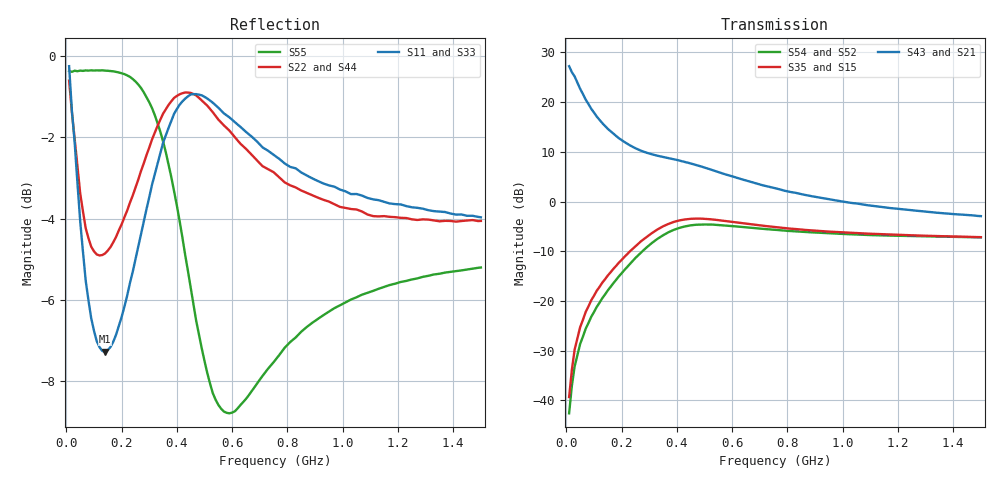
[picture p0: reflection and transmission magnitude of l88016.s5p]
!  1/8/97
!  POLYFET RF DEVICES
!  L88016
!  S PARAMETERS
!  VDS=28V, IDQ=200mA
!AWR Design Environment (2053) Wed Feb 04 14:48:35 2004
!freq-unit  param-type  data-format  keyword  impedance-ohms
# MHz  S  MA  R  50
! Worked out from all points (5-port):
!   150 points, 10 MHz to 1.5 GHz, reference 50 ohm
!   strongest paths, dB at 10 MHz, 380 MHz, 760 MHz, 1.13 GHz, 1.5 GHz:
!     S43: 27.2, 8.6, 2.6, -1.0, -2.9
!     S21: 27.2, 8.6, 2.6, -1.0, -2.9
!     S35: -39.3, -4.3, -5.2, -6.5, -7.2
!     S15: -39.3, -4.3, -5.2, -6.5, -7.2
!     S54: -42.6, -5.9, -5.7, -6.8, -7.2
!     S52: -42.6, -5.9, -5.7, -6.8, -7.2
!   lowest |S11| = -7.3 dB at 140 MHz (marker M1), VSWR 2.53, Z = 45.8 - j45.8 ohm
!   |S11| at or under -10 dB: nowhere
